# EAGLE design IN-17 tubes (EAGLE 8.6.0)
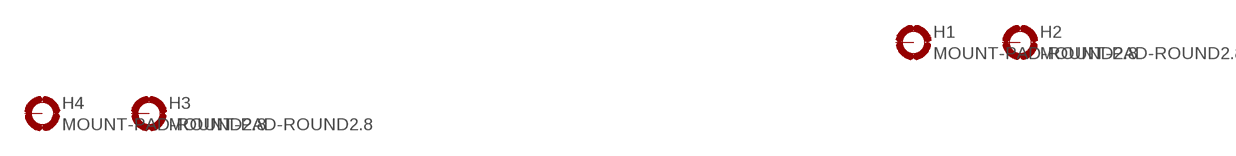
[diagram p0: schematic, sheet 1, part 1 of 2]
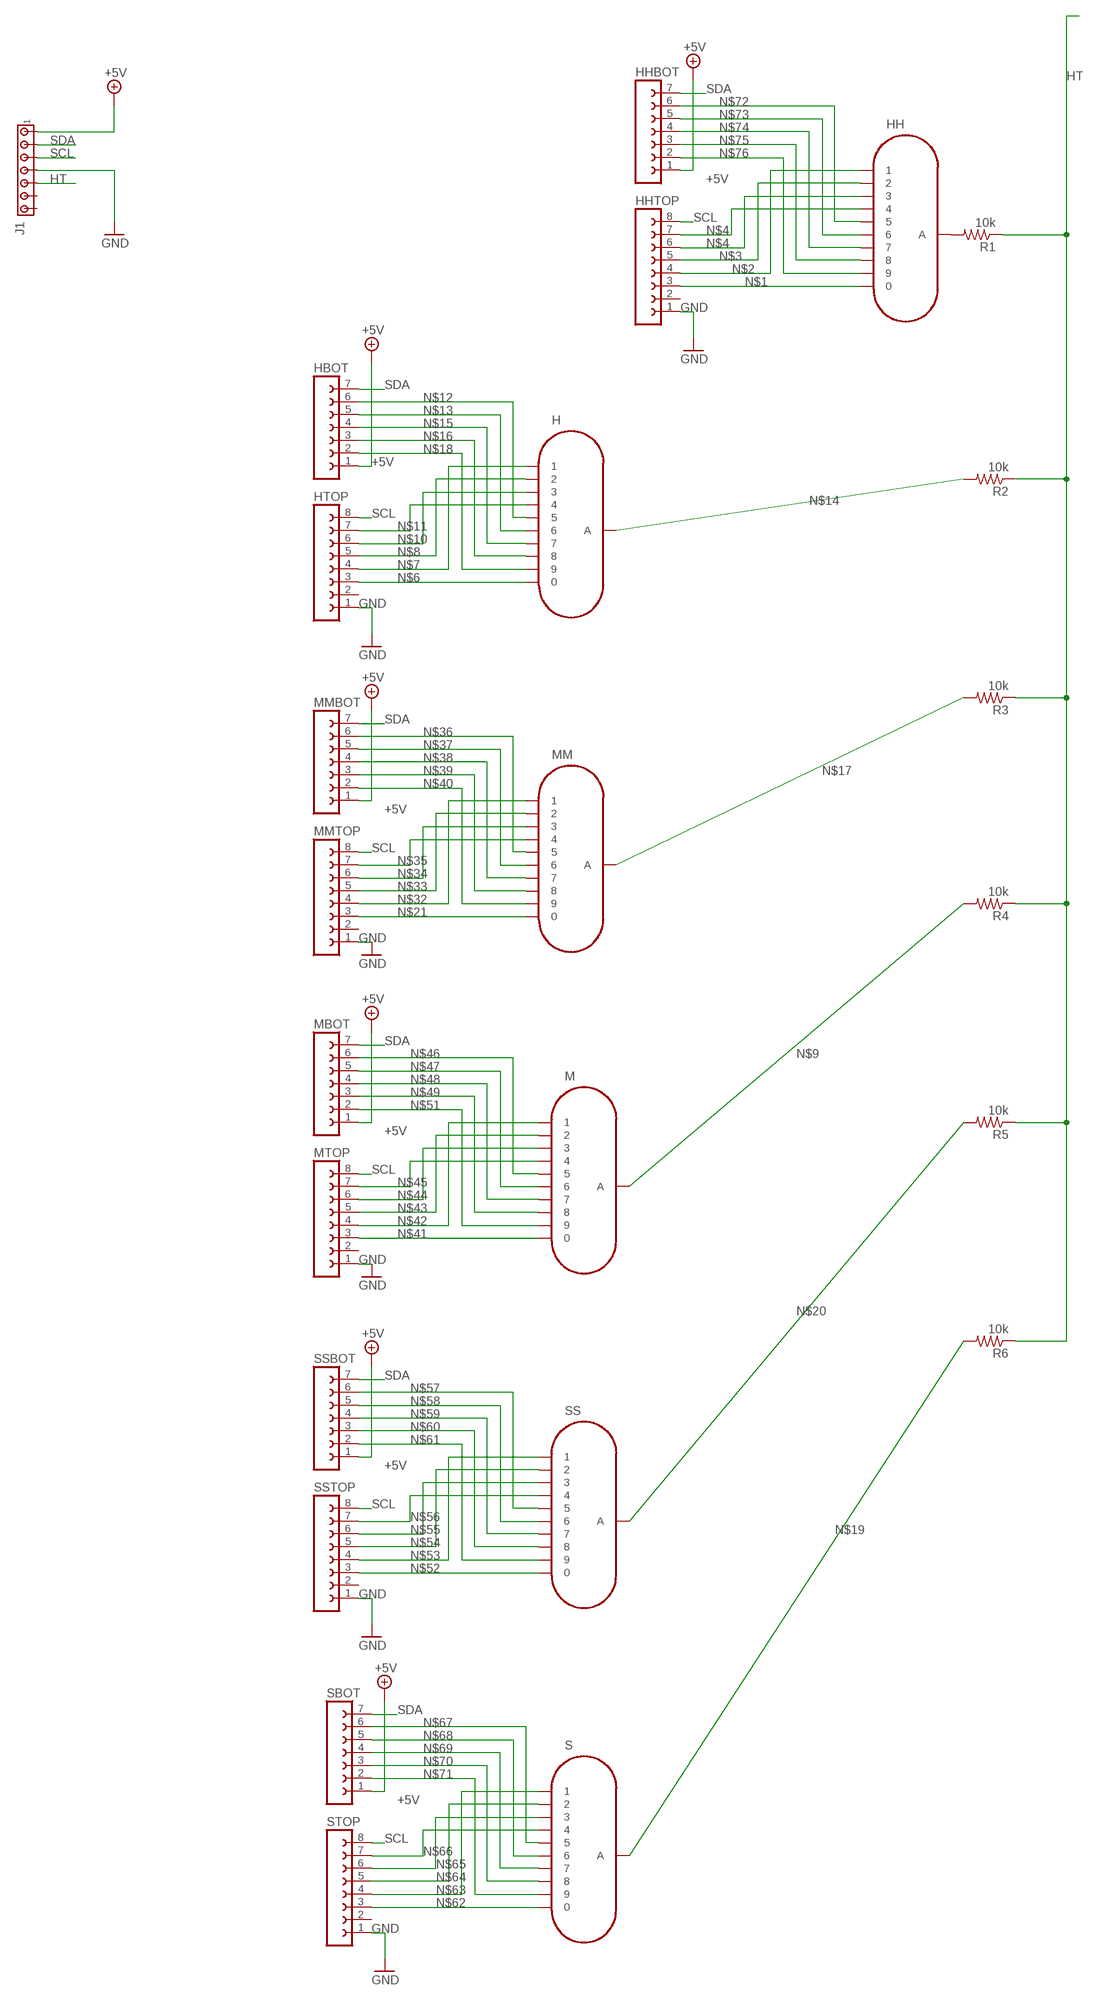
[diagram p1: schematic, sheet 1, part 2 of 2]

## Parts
H  IN-17  [IN-17]
H1  MOUNT-PAD-ROUND2.8  [2,8-PAD]
H2  MOUNT-PAD-ROUND2.8  [2,8-PAD]
H3  MOUNT-PAD-ROUND2.8  [2,8-PAD]
H4  MOUNT-PAD-ROUND2.8  [2,8-PAD]
HBOT  FE07-1  [FE07]
HH  IN-17  [IN-17]
HHBOT  FE07-1  [FE07]
HHTOP  FE08-1  [FE08]
HTOP  FE08-1  [FE08]
J1  MTA07-100  [10X07MTA]
M  IN-17  [IN-17]
MBOT  FE07-1  [FE07]
MM  IN-17  [IN-17]
MMBOT  FE07-1  [FE07]
MMTOP  FE08-1  [FE08]
MTOP  FE08-1  [FE08]
R1  10k  R-US_M0805  [M0805]
R2  10k  R-US_M0805  [M0805]
R3  10k  R-US_M0805  [M0805]
R4  10k  R-US_M0805  [M0805]
R5  10k  R-US_M0805  [M0805]
R6  10k  R-US_M0805  [M0805]
S  IN-17  [IN-17]
SBOT  FE07-1  [FE07]
SS  IN-17  [IN-17]
SSBOT  FE07-1  [FE07]
SSTOP  FE08-1  [FE08]
STOP  FE08-1  [FE08]

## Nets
+5V: HBOT.1 HHBOT.1 J1.1 MBOT.1 MMBOT.1 SBOT.1 SSBOT.1
GND: HHTOP.1 HTOP.1 J1.4 MMTOP.1 MTOP.1 SSTOP.1 STOP.1
HT: J1.5 R1.1 R2.1 R3.1 R4.1 R5.1 R6.1
N$1: HH.0 HHTOP.3
N$2: HH.1 HHTOP.4
N$3: HH.2 HHTOP.5
N$4: HH.3 HHTOP.6
N$5: HH.4 HHTOP.7
N$6: H.0 HTOP.3
N$7: H.1 HTOP.4
N$8: H.2 HTOP.5
N$9: M.A R4.2
N$10: H.3 HTOP.6
N$11: H.4 HTOP.7
N$12: H.5 HBOT.6
N$13: H.6 HBOT.5
N$14: H.A R2.2
N$15: H.7 HBOT.4
N$16: H.8 HBOT.3
N$17: MM.A R3.2
N$18: H.9 HBOT.2
N$19: R6.2 S.A
N$20: R5.2 SS.A
N$21: MM.0 MMTOP.3
N$32: MM.1 MMTOP.4
N$33: MM.2 MMTOP.5
N$34: MM.3 MMTOP.6
N$35: MM.4 MMTOP.7
N$36: MM.5 MMBOT.6
N$37: MM.6 MMBOT.5
N$38: MM.7 MMBOT.4
N$39: MM.8 MMBOT.3
N$40: MM.9 MMBOT.2
N$41: M.0 MTOP.3
N$42: M.1 MTOP.4
N$43: M.2 MTOP.5
N$44: M.3 MTOP.6
N$45: M.4 MTOP.7
N$46: M.5 MBOT.6
N$47: M.6 MBOT.5
N$48: M.7 MBOT.4
N$49: M.8 MBOT.3
N$50: HH.A R1.2
N$51: M.9 MBOT.2
N$52: SS.0 SSTOP.3
N$53: SS.1 SSTOP.4
N$54: SS.2 SSTOP.5
N$55: SS.3 SSTOP.6
N$56: SS.4 SSTOP.7
N$57: SS.5 SSBOT.6
N$58: SS.6 SSBOT.5
N$59: SS.7 SSBOT.4
N$60: SS.8 SSBOT.3
N$61: SS.9 SSBOT.2
N$62: S.0 STOP.3
N$63: S.1 STOP.4
N$64: S.2 STOP.5
N$65: S.3 STOP.6
N$66: S.4 STOP.7
N$67: S.5 SBOT.6
N$68: S.6 SBOT.5
N$69: S.7 SBOT.4
N$70: S.8 SBOT.3
N$71: S.9 SBOT.2
N$72: HH.5 HHBOT.6
N$73: HH.6 HHBOT.5
N$74: HH.7 HHBOT.4
N$75: HH.8 HHBOT.3
N$76: HH.9 HHBOT.2
SCL: HHTOP.8 HTOP.8 J1.3 MMTOP.8 MTOP.8 SSTOP.8 STOP.8
SDA: HBOT.7 HHBOT.7 J1.2 MBOT.7 MMBOT.7 SBOT.7 SSBOT.7
Unconnected: H1.B2,8(MOUNT) H2.B2,8(MOUNT) H3.B2,8(MOUNT) H4.B2,8(MOUNT) HHTOP.2 HTOP.2 J1.6 J1.7 MMTOP.2 MTOP.2 SSTOP.2 STOP.2

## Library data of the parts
H HH M MM S SS = russian-nixies:IN-17: IN-17: tiny numeric topview nixie tube
H1-H4 = holes:MOUNT-PAD-ROUND: MOUNTING PAD, round
HBOT HHBOT MBOT MMBOT SBOT SSBOT = con-lsta:FE07-1: FEMALE HEADER; OC_FARNELL: unknown; OC_NEWARK: unknown
HHTOP HTOP MMTOP MTOP SSTOP STOP = con-lsta:FE08-1: FEMALE HEADER; OC_FARNELL: unknown; OC_NEWARK: unknown
J1 = con-amp:MTA07-100: AMP connector
R1-R6 = adafruit:R-US_: RESISTOR, American symbol

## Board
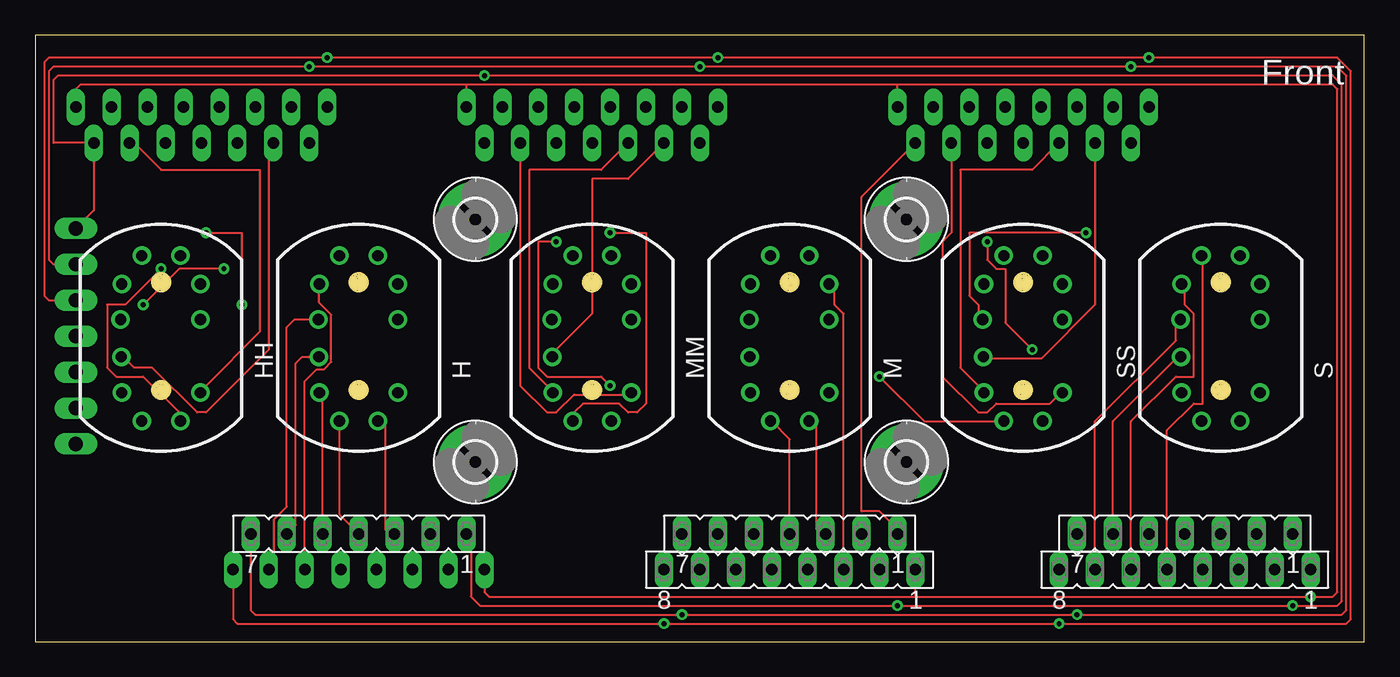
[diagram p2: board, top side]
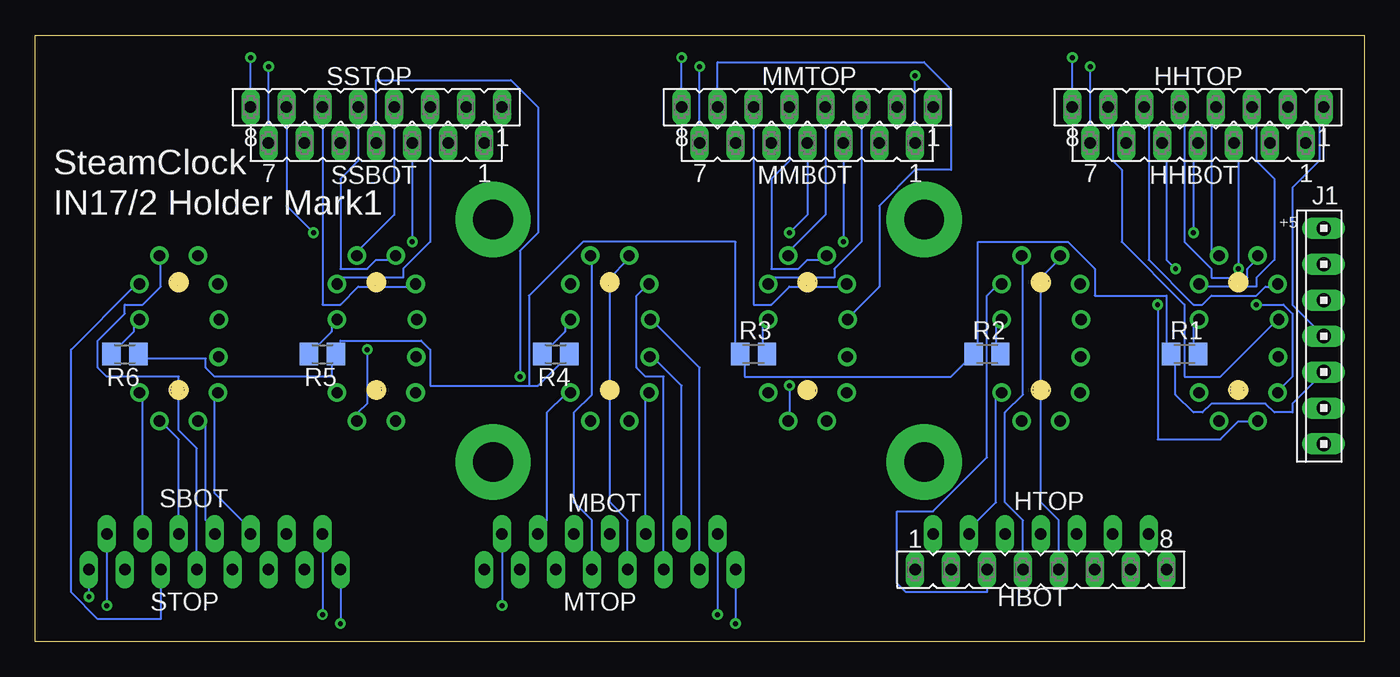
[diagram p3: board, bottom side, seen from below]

Size 93.96 x 42.85 mm. Coordinates in mm from the lower left corner, seen from the top.
Outline: 0,0 93.96,0 93.96,42.85 0,42.85 0,0
Copper layers (1*16): Top 0.035mm / dielectric 1.5mm / Bottom 0.035mm
Design rules "default": minimum track width 6mil, minimum drill 0.35mm, track to track 6mil, track to pad 6mil, pad to pad 6mil, via to via 6mil, smd to smd 6mil, copper to edge 40mil, drill to drill 6mil, minimum pad ring 10mil, minimum via ring 8mil, stop-mask expansion 4mil, vias tented up to drill 0mil, thermal gap 10mil

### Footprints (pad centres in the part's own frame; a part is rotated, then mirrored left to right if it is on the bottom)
IN-17 = drill 0.8: 0 2.777,4; 1 1.365,6; 2 -1.365,6; 3 -2.778,4; 4 -2.858,1.5; 5 -2.818,-1.143; 6 -2.778,-3.683; 7 -1.365,-5.683; 8 1.365,-5.683; 9 2.777,-3.683; A 2.777,1.5
2,8-PAD = drill 2.8 pad 5.334: B2,8 0,0
FE07 = drill 0.813 long: 1 -7.62,0; 2 -5.08,0; 3 -2.54,0; 4 0,0; 5 2.54,0; 6 5.08,0; 7 7.62,0
FE08 = drill 0.813 long: 1 -8.89,0; 2 -6.35,0; 3 -3.81,0; 4 -1.27,0; 5 1.27,0; 6 3.81,0; 7 6.35,0; 8 8.89,0
10X07MTA = drill 1.016 long: 1 7.62,0; 2 5.08,0; 3 2.54,0; 4 0,0; 5 -2.54,0; 6 -5.08,0; 7 -7.62,0
M0805 = smd 1.3 x 1.6: 1 -0.95,0; 2 0.95,0

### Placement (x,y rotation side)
H  22.86,21.27 0 top
H1  31.11,12.7 0 top
H2  61.59,12.7 0 top
H3  61.59,29.85 0 top
H4  31.11,29.85 0 top
HBOT  22.86,7.62 180 top
HH  8.89,21.27 0 top
HHBOT  11.75,35.24 180 bottom
HHTOP  11.75,37.78 180 bottom
HTOP  22.86,5.08 0 bottom
J1  2.86,21.59 90 bottom
M  53.34,21.27 0 top
MBOT  53.34,7.62 180 top
MM  39.37,21.27 0 top
MMBOT  39.37,35.24 180 bottom
MMTOP  39.37,37.78 180 bottom
MTOP  53.34,5.08 180 top
R1  12.7,20.32 0 bottom
R2  26.67,20.32 0 bottom
R3  43.18,20.32 0 bottom
R4  57.15,20.32 180 bottom
R5  73.66,20.32 180 bottom
R6  87.63,20.32 180 bottom
S  83.82,21.27 0 top
SBOT  81.28,7.62 180 top
SS  69.85,21.27 0 top
SSBOT  69.85,35.24 180 bottom
SSTOP  69.85,37.78 180 bottom
STOP  81.28,5.08 180 top

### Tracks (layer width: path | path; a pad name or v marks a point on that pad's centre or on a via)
+5V  (via drill 0.35)
  Top 0.152: HBOT.1 30.8,7.3 30.8,3.18 31.43,2.54 v60.96,2.54 v88.9,2.54 92.08,2.54 92.39,2.86 92.39,39.37 91.76,40 v31.75,40 1.59,40 1.27,39.69 1.27,35.24 HHBOT.1 4.13,30.48 J1.1 | SSBOT.1 58.42,31.43 58.42,9.21 59.69,9.21 60.96,7.94 MBOT.1
  Bottom 0.152: MBOT.1 v60.96,2.54 | SBOT.1 v88.9,2.54 | MMBOT.1 v31.75,40
GND  (via drill 0.35)
  Top 0.152: HTOP.1 31.75,3.49 32.07,3.18 62.23,3.18 | 62.23,3.18 MTOP.1 | 62.23,3.18 v90.17,3.18 91.76,3.18 92.08,3.49 92.08,39.05 91.76,39.37 60.96,39.37 | HHTOP.1 2.86,39.05 3.18,39.37 30.48,39.37 | 60.96,39.37 30.48,39.37 | MMTOP.1 30.48,39.37 | SSTOP.1 60.96,39.37
  Bottom 0.152: STOP.1 v90.17,3.18 | J1.4 5.08,23.81 5.08,32.07 3.18,33.97 3.18,37.78 HHTOP.1
HT
  Bottom 0.152: 59.06,18.1 66.04,18.1 66.04,20.64 66.67,21.27 72.39,21.27 72.39,20.64 R5.1 73.03,20 73.03,18.73 81.28,18.73 81.92,19.37 81.92,20 86.36,20 R6.1 | 59.06,18.1 58.42,18.1 56.52,20 R4.1 | J1.5 5.08,16.83 5.08,16.19 6.35,16.19 6.98,16.83 10.79,16.83 11.43,16.19 12.06,16.19 13.33,17.46 13.33,20 R1.1 13.97,20.64 13.97,24.45 19.05,24.45 19.05,26.35 20.96,28.26 27.3,28.26 27.3,20.64 R2.1 27.94,20 29.21,18.73 43.81,18.73 43.81,20 R3.1 44.45,20.64 44.45,28.26 55.25,28.26 59.06,24.45 59.06,18.1
N$1
  Bottom 0.152: HH.0 11.43,25.08 7.62,25.08 7.62,25.72 6.35,26.99 6.35,32.7 7.62,33.97 7.62,37.78 HHTOP.3
N$2
  Bottom 0.152: HH.1 10.79,27.62 10.79,37.78 HHTOP.4
N$3
  Bottom 0.152: HH.2 7.62,26.99 8.25,26.35 8.25,25.72 10.79,25.72 10.79,26.35 12.7,28.26 12.7,37.78 HHTOP.5
N$4
  Bottom 0.152: HH.3 6.35,25.08 6.98,25.08 7.62,24.45 10.79,24.45 11.43,23.81 12.06,23.81 15.24,26.99 15.24,37.78 HHTOP.6
N$5
  Bottom 0.152: HH.4 6.35,22.54 10.16,18.73 12.7,18.73 12.7,23.81 17.14,28.26 17.14,33.34 17.78,33.97 17.78,37.78 HHTOP.7
N$6
  Bottom 0.152: HTOP.3 26.67,3.49 32.39,3.49 33.02,4.13 33.02,9.21 30.48,9.21 26.67,13.02 26.67,24.45 26.04,25.08 H.0
N$7
  Bottom 0.152: HTOP.4 24.13,8.57 25.4,9.84 25.4,16.19 24.13,17.46 24.13,26.99 H.1
N$8
  Bottom 0.152: HTOP.5 21.59,8.57 22.86,9.84 22.86,25.72 21.59,26.99 H.2
N$9
  Bottom 0.152: R4.2 57.78,20.64 56.52,21.91 56.52,22.54 M.A
N$10
  Top 0.152: HTOP.6 19.05,18.41 19.88,19.25 20.41,19.25 20.93,19.76 20.93,23.1 20.08,23.94 H.3
N$11
  Top 0.152: HTOP.7 16.89,5.46 16.89,8.65 17.78,9.54 17.78,22.23 18.33,22.77 H.4
N$12
  Top 0.152: HBOT.6 18.42,8.25 18.42,19.68 18.86,20.13 H.5
N$13
  Top 0.152: HBOT.5 20.32,17.35 H.6
N$14
  Bottom 0.152: R2.2 26.04,20.64 26.04,22.54 H.A
N$15
  Top 0.152: H.7 21.5,8.99 HBOT.4
N$16
  Top 0.152: H.8 24.76,15.56 24.76,7.94 25.4,7.94 HBOT.3
N$17
  Bottom 0.152: R3.2 42.55,20.64 42.55,22.54 MM.A
N$18
  Bottom 0.152: H.9 26.04,17.46 26.04,9.84 27.94,7.94 HBOT.2
N$19
  Bottom 0.152: R6.2 88.27,20.64 87,21.91 87,22.54 S.A
N$20
  Bottom 0.152: R5.2 74.3,20.64 73.03,21.91 73.03,22.54 SS.A
N$21
  Bottom 0.152: MMTOP.3 35.56,28.26 37.47,26.35 37.47,25.72 41.91,25.72 MM.0
N$32
  Bottom 0.152: MMTOP.4 38.1,30.16 40.64,27.62 MM.1
N$33
  Bottom 0.152: MMTOP.5 40.64,33.97 41.91,32.7 41.91,26.35 40,26.35 39.37,26.99 38.1,26.99 MM.2
N$34
  Bottom 0.152: MMTOP.6 43.18,23.81 41.91,23.81 40.64,25.08 36.83,25.08 MM.3
N$35
  Bottom 0.152: MMTOP.7 45.72,40.96 31.11,40.96 29.21,39.05 29.21,33.34 31.75,33.34 34.29,30.8 34.29,25.08 36.19,23.18 MM.4
N$36
  Top 0.152: MMBOT.6 41.91,32.7 39.37,32.7 39.37,23.18 36.83,20.64 MM.5
N$37
  Top 0.152: MMBOT.5 40,33.34 34.92,33.34 34.92,19.37 36.19,18.1 MM.6
N$38  (via drill 0.35)
  Top 0.152: v40.64,28.89 43.18,28.89 43.18,16.83 42.55,16.19 41.91,16.19 41.28,16.83 38.73,16.83 38.1,16.19 MM.7
  Bottom 0.152: v40.64,28.89 39.37,30.16 MMBOT.4
N$39  (via drill 0.35)
  Top 0.152: v40.64,18.1 40,18.73 36.19,18.73 35.56,19.37 35.56,28.26 v36.83,28.26
  Bottom 0.152: v40.64,18.1 40.64,16.19 MM.8 | MMBOT.3 v36.83,28.26
N$40
  Top 0.152: MMBOT.2 34.29,18.1 36.19,16.19 36.83,16.19 38.1,17.46 41.91,17.46 MM.9
N$41
  Top 0.152: MTOP.3 57.15,23.18 56.52,23.81 56.52,25.08 M.0
N$42
  Bottom 0.152: MTOP.4 54.61,8.57 55.88,9.84 55.88,16.19 54.61,17.46 54.61,26.99 M.1
N$43
  Bottom 0.152: MTOP.5 52.07,8.57 53.34,9.84 53.34,25.72 52.07,26.99 M.2
N$44
  Bottom 0.152: MTOP.6 49.53,18.73 50.8,18.73 51.44,19.37 51.44,24.45 50.8,25.08 M.3
N$45
  Bottom 0.152: MTOP.7 46.99,19.37 50.17,22.54 M.4
N$46
  Bottom 0.152: MBOT.6 48.26,18.1 50.17,20 M.5
N$47
  Bottom 0.152: MBOT.5 50.8,17.46 M.6
N$48
  Top 0.152: MBOT.4 53.34,14.29 52.07,15.56 M.7
N$49
  Top 0.152: M.8 55.25,15.56 55.25,7.94 55.88,7.94 MBOT.3
N$50
  Bottom 0.152: R1.2 12.06,20.64 12.06,22.54 HH.A
N$51
  Bottom 0.152: M.9 56.52,17.46 57.78,16.19 57.78,8.57 58.42,7.94 MBOT.2
N$52
  Bottom 0.152: SSTOP.3 66.04,28.26 67.95,26.35 67.95,25.72 72.39,25.72 SS.0
N$53
  Bottom 0.152: SSTOP.4 68.58,30.16 71.12,27.62 SS.1
N$54
  Bottom 0.152: SSTOP.5 71.12,33.97 72.39,32.7 72.39,26.35 70.48,26.35 69.85,26.99 68.58,26.99 SS.2
N$55
  Bottom 0.152: SSTOP.6 73.66,23.81 72.39,23.81 71.12,25.08 67.31,25.08 SS.3
N$56  (via drill 0.35)
  Top 0.152: v74.3,28.89 66.04,28.89 66.04,24.45 66.67,23.81 66.67,23.18 SS.4
  Bottom 0.152: v74.3,28.89 76.2,30.8 SSTOP.7
N$57
  Top 0.152: SSBOT.6 74.93,23.81 71.12,20 67.31,20 SS.5
N$58
  Top 0.152: SSBOT.5 70.48,33.34 65.41,33.34 65.41,19.37 66.67,18.1 SS.6
N$59  (via drill 0.35)
  Top 0.152: v59.69,18.73 62.87,15.56 67.95,15.56 SS.7
  Bottom 0.152: v59.69,18.73 59.69,27.62 58.42,28.89 58.42,37.78 60.33,39.69 69.85,39.69 SSBOT.4
N$60  (via drill 0.35)
  Top 0.152: v70.48,20.64 68.58,22.54 68.58,26.35 67.95,26.35 67.31,26.99 v67.31,28.26
  Bottom 0.152: v70.48,20.64 70.48,16.83 71.12,16.19 SS.8 | SSBOT.3 v67.31,28.26
N$61
  Top 0.152: SSBOT.2 64.77,28.89 64.14,28.26 64.14,18.73 66.67,16.19 67.31,16.19 67.95,16.83 71.76,16.83 72.39,17.46 SS.9
N$62
  Bottom 0.152: STOP.3 85.09,1.59 89.53,1.59 91.44,3.49 91.44,20.64 87,25.08 S.0
N$63
  Bottom 0.152: STOP.4 82.55,13.65 83.82,14.92 83.82,18.73 88.9,18.73 89.53,19.37 89.53,21.27 87.63,23.18 87.63,23.81 86.36,23.81 85.09,25.08 85.09,26.99 S.1
N$64
  Top 0.152: STOP.5 80.01,14.92 81.92,16.83 82.55,16.83 82.55,26.99 S.2
N$65
  Top 0.152: STOP.6 77.47,15.56 80.64,18.73 81.92,18.73 81.92,23.18 81.28,23.81 81.28,25.08 S.3
N$66
  Top 0.152: STOP.7 74.93,15.56 80.64,21.27 80.64,22.54 S.4
N$67
  Top 0.152: SBOT.6 76.2,15.56 80.64,20 S.5
N$68
  Bottom 0.152: S.6 81.28,17.46 81.28,10.48 78.74,7.94 SBOT.5
N$69
  Bottom 0.152: S.7 81.92,15.56 81.92,8.57 81.28,7.94 SBOT.4
N$70
  Bottom 0.152: SBOT.3 83.82,14.29 85.09,15.56 S.8
N$71
  Bottom 0.152: SBOT.2 86.36,17.46 S.9
N$72
  Top 0.152: HH.5 6.35,20 6.98,19.37 8.25,19.37 11.43,16.19 12.06,16.19 16.51,20.64 16.51,35.24 HHBOT.6
N$73  (via drill 0.35)
  Top 0.152: v7.62,23.81 10.16,26.35 v13.33,26.35
  Bottom 0.152: v7.62,23.81 5.71,23.81 5.08,23.18 5.08,18.73 5.71,18.1 HH.6 | v13.33,26.35 13.97,26.99 13.97,35.24 HHBOT.5
N$74  (via drill 0.35)
  Top 0.152: v14.61,23.81 14.61,28.89 v12.06,28.89
  Bottom 0.152: v14.61,23.81 14.61,14.29 10.16,14.29 8.89,15.56 7.62,15.56 HH.7 | v12.06,28.89 12.06,35.24 HHBOT.4
N$75  (via drill 0.35)
  Top 0.152: v8.89,26.35 6.35,23.81 5.08,23.81 5.08,19.37 5.71,18.73 7.62,18.73 10.16,16.19 HH.8
  Bottom 0.152: v8.89,26.35 8.89,35.24 HHBOT.3
N$76
  Top 0.152: HH.9 12.06,18.1 15.87,21.91 15.87,33.34 8.89,33.34 6.98,35.24 HHBOT.2
SCL  (via drill 0.35)
  Top 0.152: HTOP.8 13.97,1.59 14.29,1.27 v44.45,1.27 v72.39,1.27 92.71,1.27 93.03,1.59 93.03,40.32 92.08,41.28 v78.74,41.28 v48.26,41.28 v20.64,41.28 0.95,41.28 0.63,40.96 0.63,24.45 0.95,24.13 J1.3
  Bottom 0.152: MTOP.8 v44.45,1.27 | STOP.8 v72.39,1.27 | SSTOP.8 v78.74,41.28 | HHTOP.8 v20.64,41.28 | MMTOP.8 v48.26,41.28
SDA  (via drill 0.35)
  Top 0.152: HBOT.7 15.24,2.22 15.56,1.91 v45.72,1.91 v73.66,1.91 92.39,1.91 92.71,2.22 92.71,40 92.08,40.64 v77.47,40.64 v46.99,40.64 v19.37,40.64 1.27,40.64 0.95,40.32 0.95,26.99 1.27,26.67 J1.2
  Bottom 0.152: MBOT.7 v45.72,1.91 | SBOT.7 v73.66,1.91 | SSBOT.7 v77.47,40.64 | HHBOT.7 v19.37,40.64 | MMBOT.7 v46.99,40.64

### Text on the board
tNames: Front
bNames: SteamClock | IN17/2 Holder Mark1 | +5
